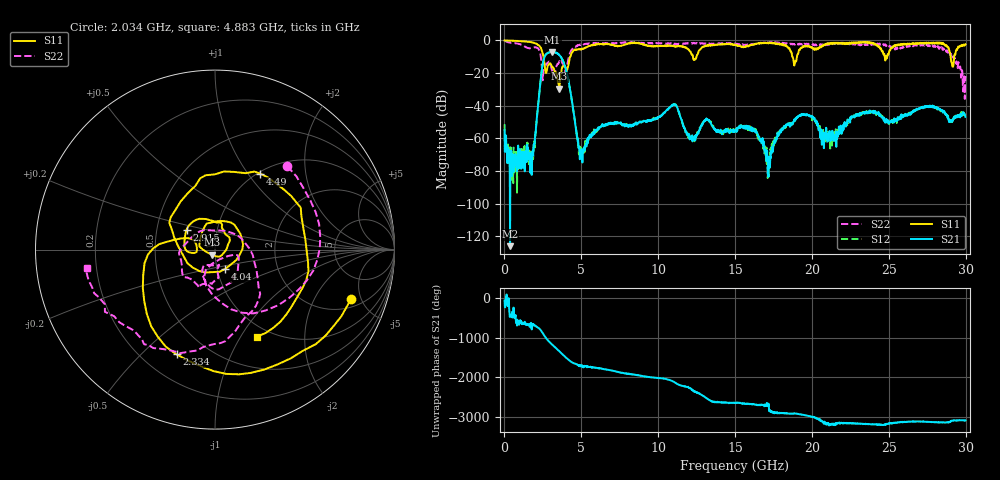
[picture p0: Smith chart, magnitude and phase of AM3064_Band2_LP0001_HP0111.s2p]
# Hz S DB R 50.0
!freq dBS11 angS11 dBS21 angS21 dBS12 angS12 dBS22 angS22
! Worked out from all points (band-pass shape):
!   1600 points, 10 MHz to 29.98 GHz, reference 50 ohm
!   highest |S21| = -7.02 dB at 3.103 GHz (marker M1); lowest = -126.1 dB at 366.1 MHz (marker M2)
!   |S21| within 3 dB of the highest: 2.613 GHz to 3.656 GHz (1.043 GHz wide, 33.3 % of centre)
!   lowest |S11| = -29.6 dB at 3.571 GHz (marker M3), VSWR 1.07, Z = 48.3 - j2.77 ohm
!   |S11| at or under -10 dB: 2.538 GHz to 4.288 GHz (1.75 GHz wide, 51.3 % of centre); 18.73 GHz to 19.02 GHz (287.9 MHz wide, 1.53 % of centre); 29.02 GHz to 29.25 GHz (228.8 MHz wide, 0.785 % of centre)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
!   |S22| runs from -35.9 to -0.2 dB; largest |S21 - S12| = 0.01
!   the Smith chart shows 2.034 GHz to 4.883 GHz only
!   S11 on the Smith chart (normalised r, x): 2.034 GHz: 2.64, -4.13; 2.334 GHz: 0.34, -0.64; 2.915 GHz: 0.71, +0.17; 4.04 GHz: 1.09, -0.24; 4.49 GHz: 1.03, +1.15; 4.883 GHz: 0.86, -1.18
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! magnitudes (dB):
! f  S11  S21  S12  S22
! 10 MHz  0.0  -55.0  -51.3  -0.2
! 366.1 MHz  -0.1  -126.1  -65.6  -1.4
! 1.716 GHz  -1.1  -73.8  -68.0  -4.7
! 2.034 GHz  -1.9  -56.3  -56.0  -4.2
! 2.334 GHz  -4.1  -26.0  -26.1  -8.4
! 2.915 GHz  -14.3  -7.4  -7.3  -13.1
! 3.103 GHz  -16.5  -7.0  -7.1  -18.8
! 3.571 GHz  -29.6  -8.9  -8.9  -12.7
! 4.04 GHz  -18.3  -19.2  -19.1  -16.7
! 4.49 GHz  -6.1  -43.6  -43.3  -4.3
! 4.883 GHz  -5.4  -67.0  -64.9  -2.8
! 5.015 GHz  -5.5  -68.5  -67.0  -2.7
! 10 GHz  -3.4  -46.9  -46.8  -1.7
! 15 GHz  -2.6  -55.8  -55.7  -1.9
! 16.34 GHz  -2.3  -56.5  -55.9  -2.2
! 17.16 GHz  -1.6  -83.7  -73.6  -1.4
! 18.08 GHz  -2.2  -54.6  -53.9  -1.5
! 19.99 GHz  -4.2  -47.0  -47.2  -2.2
! 20.76 GHz  -2.7  -59.5  -57.8  -3.1
! 25 GHz  -8.1  -51.0  -50.5  -3.0
! 28.56 GHz  -2.3  -44.0  -43.0  -4.8
! 29.98 GHz  -2.4  -46.8  -45.0  -21.8
